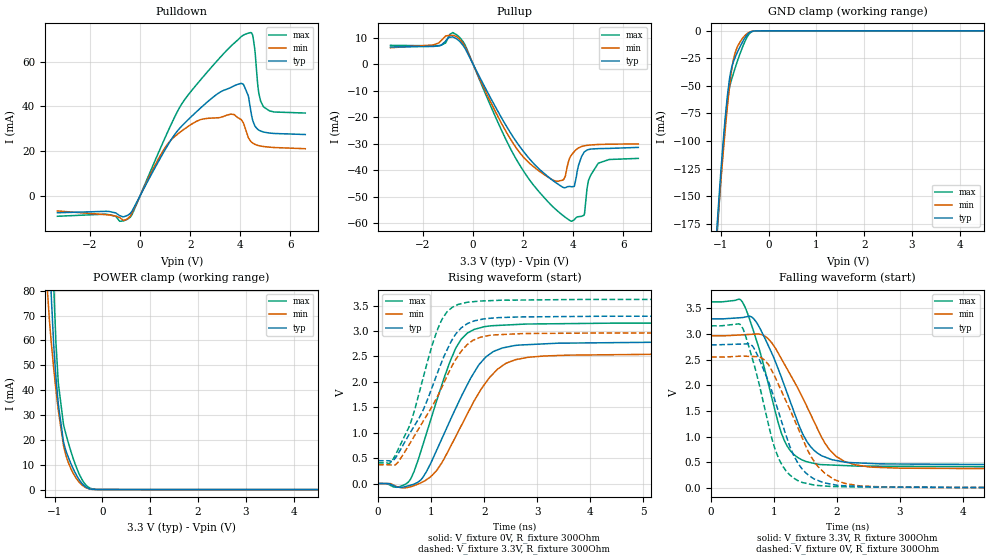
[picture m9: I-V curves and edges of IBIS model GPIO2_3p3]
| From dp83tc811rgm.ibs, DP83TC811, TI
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|   GPIO2_3p3 Model
[Model]   GPIO2_3p3
Model_type   I/O
Polarity   Non-Inverting
Enable   Active-Low
Vinl = 0.8
Vinh = 2
Vmeas = 1.65
Vref = 0
Cref = 2pF
Rref = 100000
|   typ   min   max
C_comp   3.0737pF   2.9218pF   3.1891pF
| Where Nom  PVT is Nominal Process, 3.3V, 27C
|   Fast PVT is Strong Process,  3.63V, -40C
|   Slow PVT is Weak Process,   2.97V, 125C
[Voltage Range]   3.3   2.97   3.63
|Junction Temperature
[Temperature Range]   27   125   -40
[Pullup Reference]   3.3   2.97   3.63
[Pulldown Reference]   -0   0   0
[Power Clamp Reference]   3.3   2.97   3.63
[GND Clamp Reference]   0   0   0
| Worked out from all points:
|   slope of the pulldown table from 0 to 0.495 V, typ, clamps not added: 47.3 ohm
|   slope of the pullup table from 0 to 0.495 V, typ, clamps not added: 54.4 ohm
|   GND clamp passes 1 mA (typ) near -0.38 V on its own axis
|   POWER clamp passes 1 mA (typ) near -0.35 V on its own axis
|   falling waveform, V_fixture 3.3V, R_fixture 300Ohm: 20-80 % time 544ps typ, 653ps min, 430ps max; typ from 3.3 V to 0.449 V
|   rising waveform, V_fixture 0V, R_fixture 300Ohm: 20-80 % time 776ps typ, 815ps min, 603ps max; typ from 0 V to 2.79 V
|   rising waveform, V_fixture 3.3V, R_fixture 300Ohm: 20-80 % time 730ps typ, 811ps min, 551ps max; typ from 0.449 V to 3.3 V
|   falling waveform, V_fixture 0V, R_fixture 300Ohm: 20-80 % time 486ps typ, 581ps min, 402ps max; typ from 2.79 V to 0 V
[Pulldown]
|   Voltage   I(typ)   I(min)   I(max)
-3.3V     -7.581mA   -6.781mA   -9.148mA
-399.3mV  -7.958mA   -9.17mA    -9.63mA
848.1mV   17.66mA    18.84mA    22.19mA
1.462V    28.63mA    27.26mA    37.07mA
3.63V     48.51mA    36.56mA    67mA
4.165V    49.04mA    31.46mA    72.15mA
4.323V    44.79mA    26.12mA    72.83mA
4.491V    34.15mA    23.68mA    72.11mA
4.59V     31.24mA    23.03mA    64.85mA
4.739V    29.45mA    22.47mA    46.32mA
4.927V    28.57mA    22.08mA    39.92mA
6.6V      27.44mA    21.09mA    37.05mA
[GND Clamp]
|   Voltage   I(typ)   I(min)   I(max)
-3.3V     -1.881A    -1.694A    -2.031A
-1.073V   -174.7mA   -178mA     -183.5mA
-1.023V   -143.3mA   -150.3mA   -151.1mA
-993.3mV  -125.6mA   -134.2mA   -132.3mA
-894.3mV  -73.74mA   -84.26mA   -77.09mA
-854.7mV  -56.84mA   -66.3mA    -61.32mA
-795.3mV  -38.18mA   -43.04mA   -47.74mA
-735.9mV  -28.28mA   -26.51mA   -38.9mA
-666.6mV  -20.86mA   -16.02mA   -29.49mA
-508.2mV  -7.372mA   -4.917mA   -11.04mA
-389.4mV  -1.317mA   -980.6uA   -2.142mA
6.6V      0A         0A         0A
[Pullup]
|   Voltage   I(typ)   I(min)   I(max)
-3.3V     6.512mA    6.237mA    7.137mA
-537.9mV  8.633mA    9.456mA    10.15mA
1.224V    -21.67mA   -23.88mA   -26.71mA
2.095V    -33.91mA   -35.93mA   -41.49mA
3.343V    -44.95mA   -44.22mA   -55.16mA
3.62V     -46.57mA   -43.47mA   -57.31mA
3.897V    -46.2mA    -34.69mA   -59.17mA
4.046V    -46.03mA   -32.93mA   -58.63mA
4.432V    -33.24mA   -30.82mA   -56.99mA
4.61V     -32.2mA    -30.55mA   -43.81mA
5.006V    -31.85mA   -30.29mA   -37.34mA
6.6V      -31.39mA   -30.1mA    -35.54mA
[POWER Clamp]
|   Voltage   I(typ)   I(min)   I(max)
-3.3V     2.167A     1.839A     2.428A
-1.171V   137.5mA    85.92mA    203.4mA
-1.112V   99.25mA    68.9mA     151.4mA
-1.073V   78.79mA    59.68mA    119.6mA
-1.013V   56.29mA    47.59mA    79.21mA
-973.5mV  45.41mA    40.29mA    59.47mA
-924mV    34.53mA    31.93mA    43.03mA
-815.1mV  19.17mA    17.78mA    26.17mA
-607.2mV  8.209mA    6.409mA    12.26mA
-330mV    789.8uA    620.6uA    1.52mA
-33mV     30.36uA    23.82uA    42.42uA
6.6V      0A         0A         0A
[Ramp]
R_load = 300
|   typ   min   max
dV/dt_r   1.67277/7.70967e-10   1.53312/8.12749e-10   1.89711/5.98927e-10
dV/dt_f   1.70947/5.41862e-10   1.55892/6.52921e-10   1.9329/4.28336e-10
[Falling Waveform]
V_fixture = 3.3V
V_fixture_min = 2.97V
V_fixture_max = 3.63V
R_fixture = 300Ohm
C_fixture = 0F
|   Time   V(typ)   V(min)   V(max)
0s        3.298V     2.968V     3.628V
469.7ps   3.321V     2.984V     3.669V
676.9ps   3.3V       2.998V     3.048V
900.4ps   2.799V     2.919V     2.076V
1.174ns   1.967V     2.395V     897.4mV
1.457ns   1.051V     1.757V     540.6mV
1.708ns   665.3mV    1.111V     458.7mV
2.116ns   504.5mV    519.3mV    435.5mV
3.015ns   465.2mV    383.9mV    420.9mV
20ns      448.6mV    370mV      406.2mV
[Rising Waveform]
V_fixture = 0V
V_fixture_min = 0V
V_fixture_max = 0V
R_fixture = 300Ohm
C_fixture = 0F
|   Time   V(typ)   V(min)   V(max)
0s        46uV       135.9uV    14.62uV
562.8ps   -46.83mV   -75.65mV   20.33mV
816.1ps   82.32mV    19.06mV    664.4mV
1.107ns   660.8mV    260.5mV    1.637V
1.474ns   1.502V     945.9mV    2.682V
1.685ns   1.949V     1.372V     2.96V
2.007ns   2.462V     1.95V      3.086V
2.59ns    2.716V     2.436V     3.127V
3.598ns   2.763V     2.525V     3.146V
20ns      2.788V     2.555V     3.162V
[Rising Waveform]
V_fixture = 3.3V
V_fixture_min = 2.97V
V_fixture_max = 3.63V
R_fixture = 300Ohm
C_fixture = 0F
|   Time   V(typ)   V(min)   V(max)
0s        448.6mV    370mV      406.3mV
248.7ps   438mV      363.3mV    422.8mV
574.1ps   946.1mV    745.2mV    1.092V
844ps     1.432V     1.213V     2.057V
1.039ns   1.95V      1.553V     2.783V
1.215ns   2.428V     1.921V     3.248V
1.471ns   2.95V      2.453V     3.504V
1.675ns   3.14V      2.727V     3.564V
2.739ns   3.278V     2.951V     3.61V
20ns      3.297V     2.968V     3.628V
[Falling Waveform]
|Gnd
V_fixture = 0V
V_fixture_min = 0V
V_fixture_max = 0V
R_fixture = 300Ohm
C_fixture = 0F
|   Time   V(typ)   V(min)   V(max)
0s        2.787V     2.553V     3.162V
459.6ps   2.805V     2.57V      3.191V
662.5ps   2.759V     2.563V     2.492V
854.3ps   2.249V     2.49V      1.543V
1.094ns   1.397V     1.954V     522.2mV
1.377ns   490.2mV    1.181V     143.6mV
1.65ns    169mV      497.2mV    51.77mV
2.125ns   40.85mV    87.26mV    21.14mV
2.834ns   15.44mV    13.14mV    13.91mV
20ns      48.06uV    139.3uV    14.26uV
